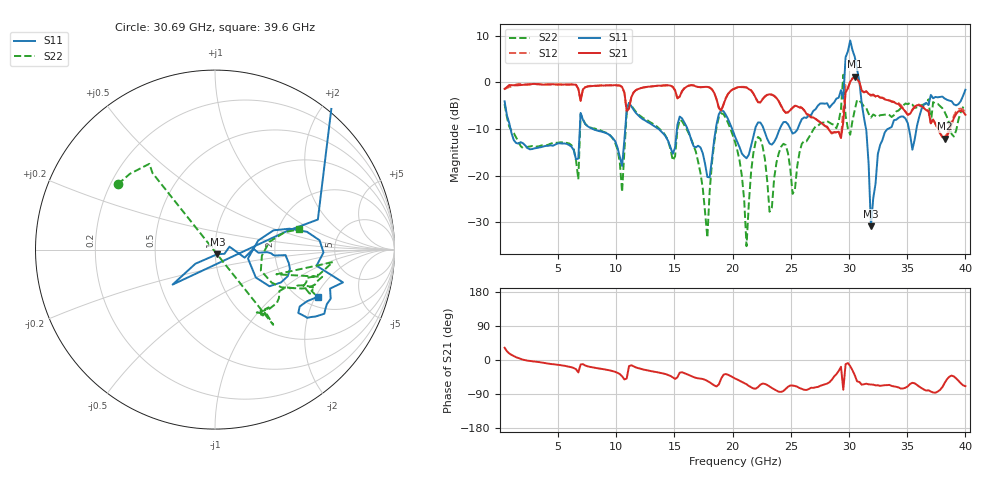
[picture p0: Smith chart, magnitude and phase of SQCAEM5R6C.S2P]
! Network Analyzer HP8722ES.07.66: Jul 25, 2000 Serial No. US39175408
! 26 Oct 2004  15:22:47
! Frequency  S11  S21  S12  S22
# HZ  S  DB R  50
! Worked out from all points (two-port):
!   201 points, 400 MHz to 40 GHz, reference 50 ohm
!   highest |S21| = 1.23 dB at 30.5 GHz (marker M1); lowest = -12.0 dB at 38.22 GHz (marker M2)
!   |S21| within 3 dB of the highest: start of sweep to 6.769 GHz; 7.108 GHz to 10.63 GHz (3.525 GHz wide, 39.7 % of centre)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
!   lowest |S11| = -30.9 dB at 31.88 GHz (marker M3), VSWR 1.06, Z = 51.3 - j2.6 ohm
!   |S11| at or under -10 dB: 915.4 MHz to 6.864 GHz (5.948 GHz wide, 153 % of centre); 8.015 GHz to 10.76 GHz (2.75 GHz wide, 29.3 % of centre); 16.13 GHz to 18.55 GHz (2.424 GHz wide, 14 % of centre)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
!   |S22| runs from -35.1 to 1.6 dB; largest |S21 - S12| = 0.18
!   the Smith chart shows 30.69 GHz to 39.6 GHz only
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4e8  -4.03 -59.8  -1.38 32.2  -1.40 36.2  -4.65 -52.2
7.132e9  -8.00 -90.1  -1.47 -11.1  -1.47 -11.8  -7.87 -101.0
1.0498e10  -17.89 -65.5  -0.96 -42.9  -0.95 -43.0  -23.47 -95.7
1.1092e10  -4.38 -71.4  -5.57 -16.2  -5.50 -15.8  -4.40 -78.5
1.3666e10  -10.03 -115.8  -0.68 -33.2  -0.69 -33.5  -9.84 -127.0
1.7824e10  -20.25 -98.6  -0.94 -55.2  -0.96 -55.2  -33.26 -54.6
1.8814e10  -6.78 -55.4  -5.39 -64.2  -5.54 -63.8  -7.37 -47.6
2.02e10  -11.58 -107.0  -1.33 -48.8  -1.23 -48.3  -12.72 -133.7
2.119e10  -16.25 -71.7  -1.06 -64.0  -1.07 -64.2  -35.09 -108.8
2.218e10  -8.57 -57.5  -4.22 -71.7  -4.24 -71.0  -11.68 -67.3
2.317e10  -13.09 -69.5  -2.53 -69.9  -2.52 -69.7  -27.72 -98.5
2.6932e10  -6.09 -43.6  -7.51 -73.5  -7.47 -72.4  -10.09 -8.9
2.9308e10  -1.65 -19.8  -11.90 -17.8  -11.80 -17.5  -5.67 -8.2
2.9506e10  -3.45 26.7  -8.49 -78.3  -5.97 -65.8  1.64 67.2
2.9704e10  5.41 -21.0  -2.17 -11.0  -0.58 -4.9  -7.11 -95.8
3.01e10  9.01 -77.1  0.18 -16.2  0.14 -15.9  -11.20 -18.3
3.0496e10  5.47 -103.7  1.23 -40.2  1.36 -38.9  -5.84 -24.4
3.0694e10  2.82 47.3  0.73 -56.5  0.86 -54.8  -3.71 146.0
3.1882e10  -30.86 -62.3  -2.67 -64.7  -2.84 -62.0  -7.53 -56.4
3.3466e10  -9.80 -5.1  -3.84 -65.7  -3.86 -64.2  -6.98 -37.3
3.8218e10  -3.44 -33.7  -12.04 -60.8  -11.64 -56.2  -6.33 -26.4
4e10  -1.57 -20.7  -6.91 -69.3  -6.38 -66.0  -4.77 -0.8
